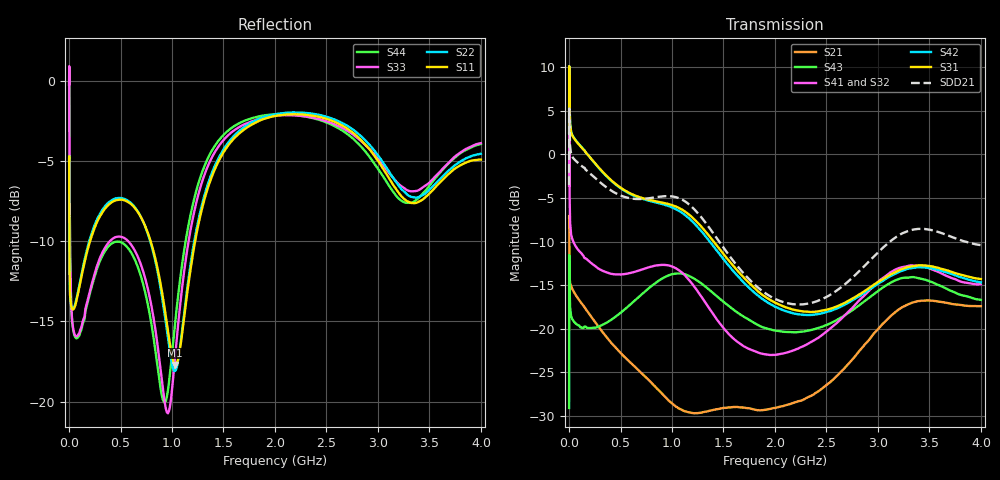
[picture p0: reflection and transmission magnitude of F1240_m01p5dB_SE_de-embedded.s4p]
! Integrated Device Technology
! Corporate Headquarters
! 6024 Silver Creek Valley Road
! San Jose, CA 95138  USA
! Phone:  1-408-284-8200
! Toll Free:  1-800-223-1366
! Webpage:  http://www.idt.com/
! Timing and RF Division
! 515 Groton Road, Suite 102
! Westford, MA 01886-6024
! Device:  F1240
! Description: Dual Intermediate Frequency Digital Variable Gain Amplifier
! Frequency:  10.0 -  500.00 MHz
! Package:  5x5 mm QFN Plastic Package: 32 pin
! Ports:  8 RF, 20 DC
!  Pin  1  = GA3 / Data  Pin 17  = RF OUT_B+
!  Pin  2  = GA4 / CLK  Pin 18  = RF OUT_B-
!  Pin  3  = GA5  Pin 19  = STBY_B
!  Pin  4  = VMODE  Pin 20  = Ground
!  Pin  5  = No Connect  Pin 21  = Ground
!  Pin  6  = GB5  Pin 22  = STB_A
!  Pin  7  = GB4  Pin 23  = RF OUT_A-  = Port 4
!  Pin  8  = GB3  Pin 24  = RF OUT_A+  = Port 3
!  Pin  9  = GB2  Pin 25  = GA0
!  Pin 10  = GB1  Pin 26  = ISET_A
!  Pin 11  = RF IN_B+  Pin 27  = VCC
!  Pin 12  = RF IN_B-  Pin 28  = Ground
!  Pin 13  = Ground  Pin 29  = RF IN_A-  = Port 2
!  Pin 14  = VCC  Pin 30  = RF IN_A+  = Port 1
!  Pin 15  = ISET_B  Pin 31  = GA1
!  Pin 16  = GB0  Pin 32  = GA2 / CSb
! Gain  = +19.5 dB
! State  = 1
! Voltage  = +5.00 V
! Current  = 85.292 mA (one channel only)
! Temperture  =  +25 C
! Test Date  =  2017-10-18
! Board  =  EB4031
! Data:  The device was measured on a custom evaluation board which has
!  individual transmission lines to the RF pins.  Data was collected
!  using a calibrated network analyzer.  The evaluation board was
!  de-embedded using Automatic Fixture Removal.
!  The reference plane is the edge of the package pin.
!  Only Channel A was measured.
!  This data is in single-ended operation.  If your needs are balanced
!  or differential S-parameters then this file needs to be used a
!  linear simulator.
! File Date:  2017-11-10  MJV
! Note:
!  Integrated Device Technology supplies this data as a sample of measured
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# Hz S dB R 100
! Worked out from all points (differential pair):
!   410 points, 500 kHz to 4 GHz, reference 100 ohm
!   strongest paths, dB at 500 kHz, 930 MHz, 1.96 GHz, 2.98 GHz, 4 GHz:
!     S31: 2.5, -5.6, -16.7, -14.8, -14.3
!     S42: 2.5, -5.8, -17.2, -15.0, -14.7
!     S41: -3.6, -12.7, -23.0, -14.9, -14.9
!     S32: -3.6, -12.9, -23.0, -15.2, -15.4
!     S43: -29.1, -14.1, -20.1, -15.9, -16.7
!     S21: -7.2, -27.8, -29.2, -20.3, -17.4
!   taken as a pair (ports 1,2 in; 3,4 out), SDD21 dB: -3.5, -4.8, -16.3, -11.5, -10.4
!   lowest |S11| = -17.7 dB at 1.03 GHz (marker M1), VSWR 1.30, Z = 78.1 - j7.79 ohm
!   |S11| at or under -10 dB: 3.374 MHz to 204.1 MHz (200.8 MHz wide, 193 % of centre); 791.9 MHz to 1.225 GHz (432.9 MHz wide, 42.9 % of centre)
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500000  -4.98 -5.6  -7.24 -5.8  -30.40 80.2  -36.33 78.3
        -7.25 -5.8  -4.98 -5.6  -36.27 77.1  -30.40 81.3
        2.46 -108.0  -3.56 -110.4  -0.26 0.6  -29.08 -43.0
        -3.59 -109.3  2.46 -106.9  -29.07 -43.2  -0.27 2.9
2000000  -6.82 -36.1  -9.73 -35.9  -20.93 29.7  -27.70 9.2
         -9.74 -36.0  -6.79 -36.2  -27.65 9.0  -20.92 29.9
         9.92 -175.2  3.25 165.6  0.02 -49.1  -11.54 -139.1
         3.20 165.9  9.93 -174.9  -11.53 -139.1  -0.03 -48.7
4000000  -10.89 -37.2  -13.58 -27.2  -21.16 9.3  -30.74 -12.6
         -13.59 -27.2  -10.87 -37.5  -30.70 -12.9  -21.15 9.4
         6.80 160.8  -2.82 138.3  -4.46 -82.7  -13.94 175.8
         -2.87 138.5  6.81 160.9  -13.93 175.7  -4.51 -82.7
1.7e8  -10.80 -102.7  -17.86 -54.7  -23.54 -43.4  -35.35 -33.3
       -17.87 -54.7  -10.63 -104.1  -35.42 -33.0  -23.55 -43.7
       0.11 116.8  -12.02 85.8  -13.95 -149.1  -19.89 108.1
       -12.00 85.6  0.12 116.0  -19.86 107.6  -14.09 -149.1
1.03e9  -17.71 -157.9  -29.26 174.1  -23.74 150.6  -31.60 -168.8
        -28.82 173.0  -18.09 -154.5  -31.57 -163.7  -24.44 150.0
        -5.95 -93.1  -13.20 169.8  -17.20 -111.7  -13.88 -126.6
        -13.01 165.7  -6.24 -95.7  -13.68 -126.7  -15.11 -107.7
2.86e9  -3.87 97.4  -22.04 -27.7  -25.34 -151.9  -27.60 -135.8
        -21.99 -27.7  -3.61 98.5  -28.42 -123.6  -26.52 -146.5
        -15.75 -64.8  -16.63 -151.2  -3.90 102.1  -17.83 -81.3
        -16.27 -161.8  -15.95 -61.8  -16.92 -79.0  -4.28 95.2
4e9  -4.93 -141.5  -17.43 105.9  -23.74 -38.5  -24.78 -22.9
     -17.40 105.8  -4.56 -139.6  -25.75 -7.8  -25.45 -31.7
     -14.29 44.2  -15.35 -58.6  -3.90 -133.8  -18.21 65.9
     -14.88 -71.8  -14.67 50.2  -16.67 57.6  -3.95 -143.6
